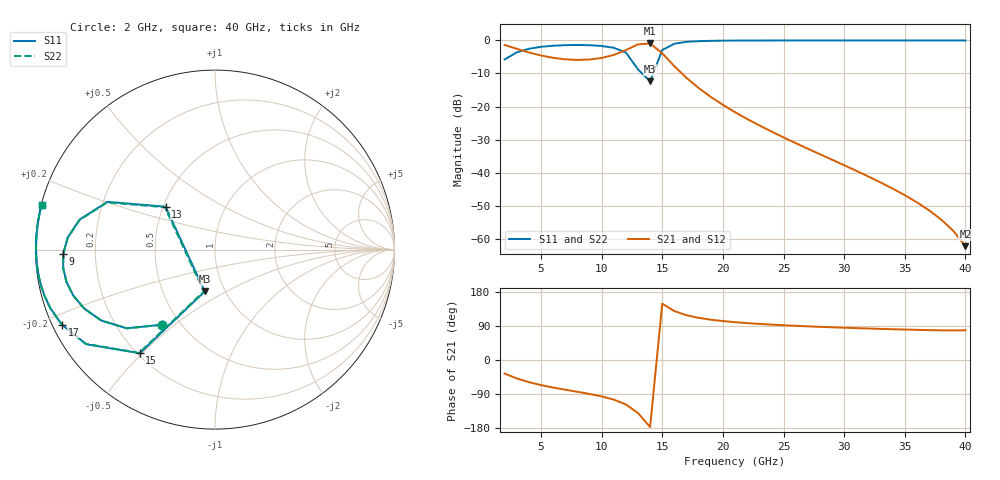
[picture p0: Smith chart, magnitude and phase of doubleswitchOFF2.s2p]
# GHZ S RI R 50
!Output file by Shape3_31
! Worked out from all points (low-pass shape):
!   39 points, 2 GHz to 40 GHz, reference 50 ohm
!   highest |S21| = -0.93 dB at 14 GHz (marker M1); lowest = -62.2 dB at 40 GHz (marker M2)
!   |S21| within 3 dB of the highest: start of sweep to 4.307 GHz; 11.32 GHz to 15.01 GHz (3.689 GHz wide, 28 % of centre)
!   lowest |S11| = -12.4 dB at 14 GHz (marker M3), VSWR 1.63, Z = 40.2 - j19.9 ohm
!   |S11| at or under -10 dB: 13.34 GHz to 14.25 GHz (911 MHz wide, 6.6 % of centre)
!   |S22| runs from -12.3 to 0.0 dB; largest |S21 - S12| = 1.1e-14
!   S11 on the Smith chart (normalised r, x): 2 GHz: 0.40, -0.45; 9 GHz: 0.08, -0.01; 13 GHz: 0.51, +0.28; 15 GHz: 0.21, -0.49; 17 GHz: 0.03, -0.23; 40 GHz: 0.00, +0.13
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2  -0.298 -0.4188  0.6911 -0.4989  0.6911 -0.4989  -0.2978 -0.4189
3  -0.4912 -0.4386  0.4931 -0.5595  0.4931 -0.5595  -0.491 -0.4388
4  -0.6332 -0.3952  0.3441 -0.5598  0.3441 -0.5598  -0.633 -0.3957
5  -0.7287 -0.3284  0.2386 -0.5406  0.2386 -0.5406  -0.7284 -0.329
7  -0.8276 -0.1796  0.104 -0.5069  0.104 -0.5069  -0.8275 -0.1807
9  -0.8454 -0.0222  0.00416 -0.5134  0.00416 -0.5134  -0.8454 -0.0238
10  -0.8209 0.0667  -0.0571 -0.5393  -0.0571 -0.5393  -0.8212 0.0647
11  -0.7546 0.1671  -0.1511 -0.5837  -0.1511 -0.5837  -0.7553 0.1646
12  -0.5993 0.2662  -0.3273 -0.6325  -0.3273 -0.6325  -0.6009 0.2631
13  -0.2756 0.2391  -0.6666 -0.5605  -0.6666 -0.5605  -0.2792 0.2361
14  -0.0573 -0.2332  -0.8971 -0.0488  -0.8971 -0.0488  -0.0625 -0.2334
15  -0.4193 -0.5776  -0.5462 0.3318  -0.5462 0.3318  -0.4227 -0.5755
16  -0.7178 -0.5272  -0.2567 0.3158  -0.2567 0.3158  -0.7194 -0.5252
17  -0.8533 -0.4183  -0.1278 0.239  -0.1278 0.239  -0.8542 -0.4168
19  -0.9507 -0.2558  -0.0395 0.1342  -0.0395 0.1342  -0.9509 -0.2551
21  -0.9812 -0.1516  -0.014 0.0809  -0.014 0.0809  -0.9812 -0.1514
28  -0.9959 0.0538  0.000817 0.019  0.000817 0.019  -0.9959 0.0531
34  -0.9841 0.1636  0.000877 0.00567  0.000877 0.00567  -0.9843 0.1625
36  -0.9785 0.1943  0.000644 0.0035  0.000644 0.0035  -0.9788 0.1931
38  -0.9724 0.223  0.000396 0.00192  0.000396 0.00192  -0.9727 0.2217
39  -0.9692 0.2367  0.000273 0.00129  0.000273 0.00129  -0.9695 0.2354
40  -0.9658 0.25  0.000154 0.000757  0.000154 0.000757  -0.9662 0.2486
